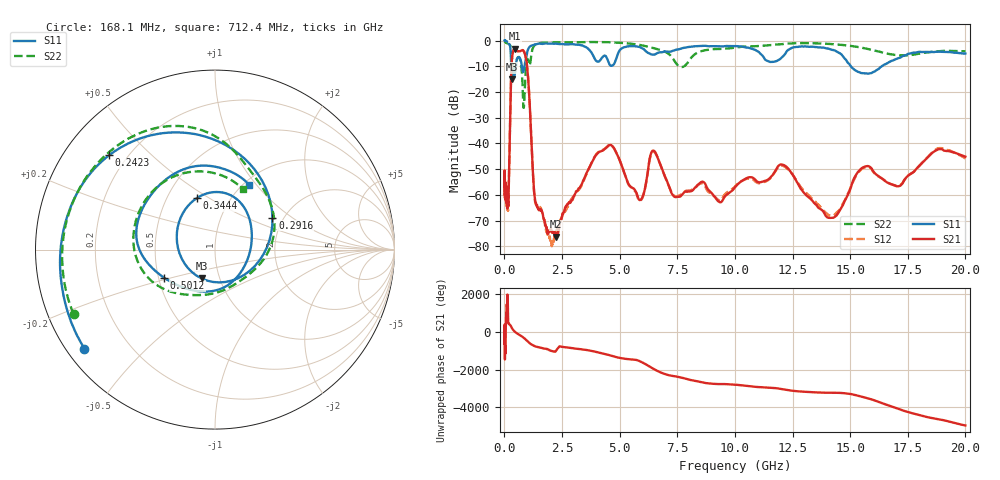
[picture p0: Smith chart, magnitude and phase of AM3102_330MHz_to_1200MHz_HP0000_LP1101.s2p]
! Date/Time: Tue, Sep 11, 2018 5:09 PM
! Network Analyzer: Agilent Technologies E8362B Rev: A.07.50.63
! Sweep from 0.010 to 20.000 GHz, 1601 Points, Sweep Type: LOG
! Power Supply: 4.950 V, 0.001 A
# Hz S DB R 50
!freq MagS11 AngS11 MagS21 AngS21 MagS12 AngS12 MagS22 AngS22
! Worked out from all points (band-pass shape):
!   1601 points, 10 MHz to 20 GHz, reference 50 ohm
!   highest |S21| = -3.19 dB at 464.5 MHz (marker M1); lowest = -76.2 dB at 2.228 GHz (marker M2)
!   |S21| within 3 dB of the highest: 335.3 MHz to 921.5 MHz (586.2 MHz wide, 93.3 % of centre)
!   lowest |S11| = -15.0 dB at 314.7 MHz (marker M3), VSWR 1.43, Z = 41 - j13.6 ohm
!   |S11| at or under -10 dB: 362.2 MHz to 498.7 MHz (136.4 MHz wide, 31.7 % of centre); 759.2 MHz to 869.9 MHz (110.7 MHz wide, 13.6 % of centre); 15.03 GHz to 16.37 GHz (1.348 GHz wide, 8.58 % of centre)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
!   |S22| runs from -26.2 to -0.3 dB; largest |S21 - S12| = 0.012
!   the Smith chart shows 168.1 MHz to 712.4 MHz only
!   S11 on the Smith chart (normalised r, x): 168.1 MHz: 0.05, -0.34; 242.3 MHz: 0.13, +0.38; 291.6 MHz: 1.75, +0.72; 344.4 MHz: 0.70, +0.44; 501.2 MHz: 0.54, -0.19; 712.4 MHz: 1.06, +0.92
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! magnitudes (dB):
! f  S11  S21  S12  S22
! 10 MHz  0.0  -51.3  -55.1  -0.3
! 35.55 MHz  0.0  -59.7  -61.2  -0.6
! 126.4 MHz  -0.4  -64.7  -63.3  -1.1
! 168.1 MHz  -0.8  -62.5  -63.7  -1.2
! 242.3 MHz  -2.0  -34.3  -34.3  -1.8
! 291.6 MHz  -8.7  -13.8  -13.9  -3.4
! 314.7 MHz  -15.0  -8.3  -8.3  -5.5
! 344.4 MHz  -10.3  -5.7  -5.7  -7.5
! 447.2 MHz  -13.2  -3.2  -3.2  -12.4
! 464.5 MHz  -12.4  -3.2  -3.2  -11.6
! 501.2 MHz  -9.8  -3.3  -3.5  -9.5
! 712.4 MHz  -7.8  -4.0  -4.1  -8.6
! 837.2 MHz  -11.6  -4.1  -4.1  -26.2
! 979.3 MHz  -4.9  -9.7  -9.7  -7.8
! 1.309 GHz  -1.6  -60.4  -61.0  -1.8
! 1.59 GHz  -1.3  -66.0  -65.3  -0.9
! 2.228 GHz  -1.2  -76.2  -74.5  -0.7
! 4.479 GHz  -7.5  -41.2  -41.1  -0.6
! 5.652 GHz  -2.2  -58.0  -58.4  -1.4
! 12.09 GHz  -6.1  -48.3  -48.7  -1.3
! 14.14 GHz  -3.4  -68.9  -68.0  -1.3
! 20 GHz  -5.0  -45.1  -45.8  -4.2
